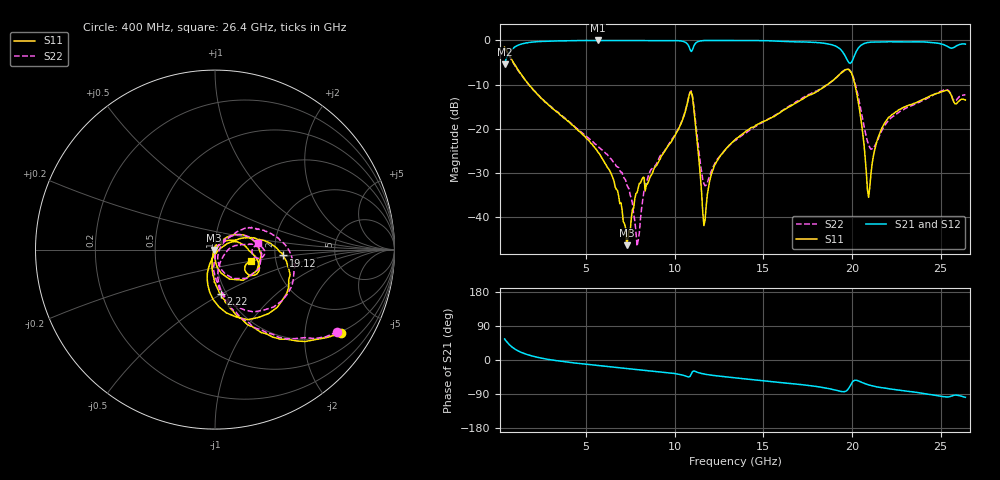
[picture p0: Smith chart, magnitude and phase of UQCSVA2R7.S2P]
!  Part Number  UQCSVA2R7  Mounting Orientation: Horizontal
!  Description: Ultra Low ESR Microwave capacitors
!  Application: Coupling, Bypass, Tuning, DC Block
!  Filters, Matching
# GHZ S DB R 50
! Freq  |S11|  S11 Ph  |S21|  S21 Ph  |S12|  S12 Ph  |S22|  S22 Ph
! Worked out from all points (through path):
!   401 points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, 400 MHz to 26.4 GHz, reference 50 ohm
!   highest |S21| = 0.00 dB at 5.665 GHz (marker M1); lowest = -5.4 dB at 400 MHz (marker M2)
!   group delay of S21, straight-line fit = 12.1 ps
!   lowest |S11| = -46.4 dB at 7.29 GHz (marker M3), VSWR 1.01, Z = 49.6 - j0.173 ohm
!   |S11| at or under -10 dB: 1.769 GHz to 18.62 GHz (16.85 GHz wide, 165 % of centre); 20.17 GHz to end of sweep
!   |S22| runs from -46.6 to -1.7 dB; largest |S21 - S12| = 0.016
!   S11 on the Smith chart (normalised r, x): 400 MHz: 0.96, -3.03; 2.22 GHz: 0.94, -0.49; 19.12 GHz: 2.21, -0.17; 26.4 GHz: 1.49, -0.20
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0.4  -1.51 -33.6  -5.37 55.6  -5.53 55.7  -1.72 -33.9
1.115  -6.41 -64.1  -1.16 25.2  -1.27 25.4  -6.51 -64.1
2.22  -12.08 -82.6  -0.29 7.4  -0.29 8.2  -12.01 -80.9
4.755  -21.10 -100.4  -0.02 -10.1  -0.01 -10.0  -20.85 -93.9
5.665  -25.29 -106.3  0.00 -14.8  -0.01 -14.8  -23.95 -92.3
6.445  -30.49 -114.4  -0.01 -18.6  -0.04 -18.6  -27.02 -90.6
7.29  -46.41 -158.5  -0.01 -22.5  -0.01 -22.3  -32.64 -92.7
7.94  -33.37 80.1  -0.01 -25.5  -0.01 -25.6  -45.24 154.6
8.395  -32.84 48.6  0.00 -27.7  -0.01 -27.8  -32.26 52.4
9.11  -27.30 53.7  0.00 -30.9  -0.01 -31.0  -26.66 50.6
10.93  -11.65 -26.8  -2.52 -37.5  -2.44 -37.6  -11.41 -22.9
11.71  -40.71 10.6  0.00 -37.5  0.00 -37.6  -32.92 -19.9
12.23  -28.35 45.1  -0.01 -41.0  -0.01 -41.2  -28.10 28.9
13.4  -22.52 39.1  -0.01 -47.0  -0.01 -47.0  -22.68 40.2
17.755  -12.15 13.0  -0.42 -68.5  -0.41 -68.8  -11.87 27.2
19.12  -8.39 -4.9  -1.37 -80.0  -1.42 -80.1  -8.40 6.0
19.64  -6.59 -31.4  -3.70 -82.5  -3.76 -82.5  -6.62 -20.6
20.095  -8.91 -79.8  -3.89 -54.9  -3.89 -54.9  -8.51 -63.7
20.94  -35.53 -36.0  -0.45 -65.7  -0.48 -65.6  -23.58 -55.6
21.46  -22.19 26.3  -0.35 -71.4  -0.38 -71.1  -22.58 0.2
22.11  -17.29 17.3  -0.31 -76.0  -0.31 -75.8  -17.94 11.1
26.4  -13.48 -17.6  -0.83 -98.6  -0.78 -98.5  -12.34 8.7
